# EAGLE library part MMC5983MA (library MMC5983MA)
3-AXIS MAGNETIC SENSOR Source: Datasheet
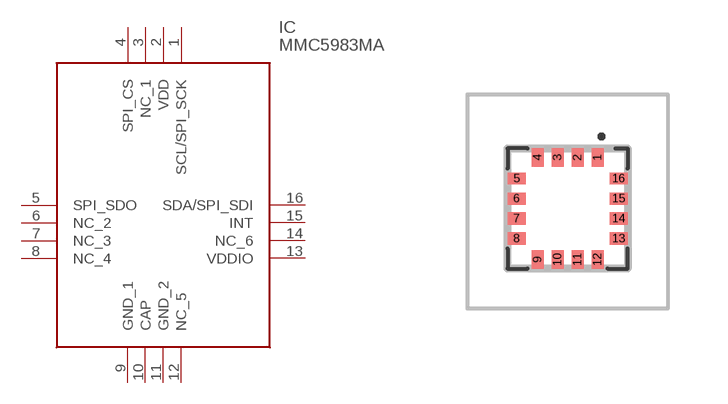
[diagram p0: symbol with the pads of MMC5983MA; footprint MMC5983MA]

Designator prefix IC

## MMC5983MA (Arrow_Part_Number: MMC5983MA; Arrow_Price-Stock: https://www.arrow.com/en/products/mmc5983ma/memsic?utm_currency=USD&region=nac; Description: 3-AXIS MAGNETIC SENSOR; Height: 1mm; Manufacturer_Name: MEMSIC; Manufacturer_Part_Number: MMC5983MA; Mouser_Part_Number: 438-MMC5983MA; Mouser_Price-Stock: https://www.mouser.co.uk/ProductDetail/MEMSIC/MMC5983MA?qs=B6kkDfuK7%2FD5qasHMdEt2g%3D%3D)  [MMC5983MA]
1  SCL/SPI_SCK
2  VDD
3  NC_1
4  SPI_CS
5  SPI_SDO
6  NC_2
7  NC_3
8  NC_4
9  GND_1
10  CAP
11  GND_2
12  NC_5
13  VDDIO
14  NC_6
15  INT
16  SDA/SPI_SDI

## Footprint MMC5983MA (pad centres in mm)
MMC5983MA-7
smd 0.3 x 0.45: 1 0.75,1.275; 2 0.25,1.275; 3 -0.25,1.275; 4 -0.75,1.275; 9 -0.75,-1.275; 10 -0.25,-1.275; 11 0.25,-1.275; 12 0.75,-1.275
smd 0.45 x 0.3: 5 -1.275,0.75; 6 -1.275,0.25; 7 -1.275,-0.25; 8 -1.275,-0.75; 13 1.275,-0.75; 14 1.275,-0.25; 15 1.275,0.25; 16 1.275,0.75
